PROGRAM MAIN
VAR CONSTANT
    cInitSource			: ST_MA_MultiArray_InitPars 
							:= ( eTypeCode := eMA_TypeCode_LREAL, nDims := 2, aDimSizes := [cChannels, cBufferLength]);
END_VAR

VAR
	(* Input *)	
	nInputSelection			: UDINT := 1;						// Switch between hardware and function generator	
	nSample					: UDINT;							// local variable
	// Hardware
	aEl3632Ch1 AT %I*		: ARRAY[1..cOversamples] OF INT;	// Input from hardware e.g. EL3632 ch1
	aEl3632Ch2 AT %I*		: ARRAY[1..cOversamples] OF INT;	// Input from hardware e.g. EL3632 ch2
	// Function generator
	fbFunctionGenerator1	: FB_FunctionGenerator;				// Signal Generator, ch1
	fSetFrequency1			: LREAL := 400;						// Hz
	fSetAmplitude1			: LREAL := 4;						// peak amplitude of sin signal [m/s^2]
	fbFunctionGenerator2	: FB_FunctionGenerator;				// Signal Generator, ch2
	fSetFrequency2			: LREAL := 35;						// Hz
	fSetAmplitude2			: LREAL := 4;						// peak amplitude of sin signal	[m/s^2]	
	fAmplitudeNoise         : LREAL;
	// additive noise for generated signals
	fbRand					: DRAND;                          	// random number generator
	fRandomNumber			: LREAL;							// value of noise
	fVar					: LREAL := 15;						// variance of added noise
		
	(* Input from aBuffer to fbSource *)
	aBuffer				: ARRAY[1..cChannels] OF ARRAY[1..cOversamples] OF LREAL;						
	fbSource			: FB_CMA_Source :=(	stInitPars := cInitSource, nOwnID := eID_Source, aDestIDs := [eID_IntegratedRMS]);
										
	(* From fbSink to aRMSResult *)	
	aRMSResult   		: ARRAY[1..cChannels] OF ARRAY[0..cOrderRMS] OF LREAL;	// Copy result
	fbIntRMS_Sink		: FB_CMA_Sink := (nOwnID := eID_IntegratedRMS_Sink);
	
	(* From fbMean_Sink to aRMSMean *)
	aRMSMean	    	: ARRAY[1..cChannels] OF ARRAY[0..cOrderRMS] OF LREAL;	// Copy result
	fbMean_Sink			: FB_CMA_Sink := (nOwnID := eID_EmpiricalMean_Sink);

	(* From fbStd_Sink to aRMSStd *)
	aRMSStd	    		: ARRAY[1..cChannels] OF ARRAY[0..cOrderRMS] OF LREAL;	// Copy result
	fbStd_Sink			: FB_CMA_Sink := (nOwnID := eID_EmpiricalStd_Sink);
	
	(* From fbClass_Sink to aClass *)	
	aClass				: ARRAY[1..cChannels] OF ARRAY[0..cOrderRMS] OF DINT;	// Copy result									
	fbClass_Sink		: FB_CMA_Sink := (nOwnID := eID_Classify_Sink);		
	
	(* Classify calculated RMS values *)
	nCountResults		: ULINT;
	bCalculate			: BOOL;
	bCalculateStat		: BOOL;
	bCalculateClass		: BOOL;
	ISOClassIs_Acc		: ARRAY[1..cChannels] OF E_IsoClass;
	ISOClassIs_Vel		: ARRAY[1..cChannels] OF E_IsoClass;
	ISOClassIs_Displ	: ARRAY[1..cChannels] OF E_IsoClass;
	
	(* little helper variables *)
	nChannel			: UDINT;
	Channel1			: ST_Channel;
	Channel2			: ST_Channel;
	
	(* output *)
	ISO_10816_Classification AT%Q* : E_IsoClass := E_IsoClass.N;

END_VAR

(* Generate input signals *)
MAIN.InputSignal();			

(* Call source to collect data *)
fbSource.Input2DStd(pDataIn 		:= ADR(aBuffer),
					nDataInSize 	:= SIZEOF(aBuffer), 
					eElementType	:= eMA_TypeCode_LREAL,
					nOptionPars		:= cCMA_Option_MarkInterruption ); 
IF fbSource.bError THEN
	fbErrHist.AddError(bErr:=TRUE, hrErrCode:=fbSource.hrErrorCode, sErrSource:='MAIN.fbSource.Input2DStd()'); // error monitoring
	// ToDo: if error
END_IF

(* Call Sinks to get results back to this task *)
MAIN.CallSinks();

(* Calculate results, i.e. determine classification *)
MAIN.CalculateResults();

ACTION CalculateResults:
// results of RMS calculation 
IF bCalculate THEN
	// channel 1
	Channel1.AccRMS   := aRMSResult[1][0];
	Channel1.VelRMS   := aRMSResult[1][1];
	Channel1.DispRMS  := aRMSResult[1][2];
	// channel 2
	Channel2.AccRMS   := aRMSResult[2][0];
	Channel2.VelRMS   := aRMSResult[2][1];
	Channel2.DispRMS  := aRMSResult[2][2];	
END_IF

// results of RMS statistics
IF bCalculateStat THEN
	// channel 1
	Channel1.AccMeanRMS				:= aRMSMean[1][0];
	Channel1.AccStdRMS				:= aRMSStd[1][0];
	Channel1.AccMeanPlusStdRms		:= Channel1.AccMeanRMS + Channel1.AccStdRMS;
	Channel1.AccMeanMinusStdRms		:= Channel1.AccMeanRMS - Channel1.AccStdRMS;
	Channel1.VelMeanRMS				:= aRMSMean[1][1];
	Channel1.VelStdRMS				:= aRMSStd[1][1];
	Channel1.VelMeanPlusStdRms		:= Channel1.VelMeanRMS + Channel1.VelStdRMS;
	Channel1.VelMeanMinusStdRms		:= Channel1.VelMeanRMS - Channel1.VelStdRMS;
	Channel1.DispMeanRMS			:= aRMSMean[1][2];
	Channel1.DispStdRMS				:= aRMSStd[1][2];
	Channel1.DispMeanPlusStdRms		:= Channel1.DispMeanRMS + Channel1.DispStdRMS;
	Channel1.DispMeanMinusStdRms	:= Channel1.DispMeanRMS - Channel1.DispStdRMS;
	
	// channel 2
	Channel2.AccMeanRMS				:= aRMSMean[2][0];
	Channel2.AccStdRMS				:= aRMSStd[2][0];
	Channel2.AccMeanPlusStdRms		:= Channel2.AccMeanRMS + Channel2.AccStdRMS;
	Channel2.AccMeanMinusStdRms		:= Channel2.AccMeanRMS - Channel2.AccStdRMS;
	Channel2.VelMeanRMS				:= aRMSMean[2][1];
	Channel2.VelStdRMS				:= aRMSStd[2][1];
	Channel2.VelMeanPlusStdRms		:= Channel2.VelMeanRMS + Channel2.VelStdRMS;
	Channel2.VelMeanMinusStdRms		:= Channel2.VelMeanRMS - Channel2.VelStdRMS;
	Channel2.DispMeanRMS			:= aRMSMean[2][2];
	Channel2.DispStdRMS				:= aRMSStd[2][2];
	Channel2.DispMeanPlusStdRms		:= Channel2.DispMeanRMS + Channel2.DispStdRMS;
	Channel2.DispMeanMinusStdRms	:= Channel2.DispMeanRMS - Channel2.DispStdRMS;
END_IF

// results of classification
IF bCalculateClass THEN
	nCountResults := nCountResults + 1;
	
	// do for each channel, shift classification results, i.e. convert range [-2..cMaxClasses-1] to [0..cMaxClasses+1]
	FOR nChannel := 1 TO cChannels DO
		ISOClassIs_Acc[nChannel]	:= DINT_TO_UDINT(aClass[nChannel][0] + 2);
		ISOClassIs_Vel[nChannel]	:= DINT_TO_UDINT(aClass[nChannel][1] + 2);
		ISOClassIs_Displ[nChannel]	:= DINT_TO_UDINT(aClass[nChannel][2] + 2);
	END_FOR
	
	// according to ISO 10816-3 select worst case 		
	ISO_10816_Classification := E_IsoClass.A;
	FOR  nChannel := 1 TO cChannels DO
		IF ISOClassIs_Acc[nChannel] > ISO_10816_Classification THEN
			ISO_10816_Classification := ISOClassIs_Acc[nChannel];
		END_IF
		IF ISOClassIs_Vel[nChannel] > ISO_10816_Classification THEN
			ISO_10816_Classification := ISOClassIs_Vel[nChannel];
		END_IF
		IF ISOClassIs_Displ[nChannel] > ISO_10816_Classification THEN
			ISO_10816_Classification := ISOClassIs_Displ[nChannel];
		END_IF
	END_FOR;

END_IF
END_ACTION

ACTION CallSinks:
(* Push results to sink *)
fbIntRMS_Sink.Output2DStd(	pDataOut 		:= ADR(aRMSResult), 
							nDataOutSize 	:= SIZEOF(aRMSResult), 
							eElementType 	:= eMA_TypeCode_LREAL, 
							nOptionPars		:= 0,
							bNewResult		=> bCalculate);
IF fbIntRMS_Sink.bError THEN
	fbErrHist.AddError(bErr:=TRUE, hrErrCode:=fbIntRMS_Sink.hrErrorCode, sErrSource:='MAIN.fbIntRMS_Sink.Output2DStd()'); // error monitoring
	// ToDo: if error
END_IF

(* Sink of mean of RMS *)
fbMean_Sink.Output2DStd(	pDataOut 		:= ADR(aRMSMean), 
							nDataOutSize 	:= SIZEOF(aRMSMean), 
							eElementType 	:= eMA_TypeCode_LREAL, 
							nOptionPars		:= 0,
							bNewResult		=> bCalculateStat);
IF fbMean_Sink.bError THEN
	fbErrHist.AddError(bErr:=TRUE, hrErrCode:=fbMean_Sink.hrErrorCode, sErrSource:='MAIN.fbMean_Sink.Output2DStd()'); // error monitoring
	// ToDo: if error
END_IF

(* Sink of standard deviation of RMS *)
fbStd_Sink.Output2DStd(	pDataOut 		:= ADR(aRMSStd), 
						nDataOutSize 	:= SIZEOF(aRMSStd), 
						eElementType 	:= eMA_TypeCode_LREAL, 
						nOptionPars		:= 0,
						bNewResult		=> bCalculateStat);
IF fbStd_Sink.bError THEN
	fbErrHist.AddError(bErr:=TRUE, hrErrCode:=fbStd_Sink.hrErrorCode, sErrSource:='MAIN.fbStd_Sink.Output2DStd()'); // error monitoring
	// ToDo: if error
END_IF

(* Sink classification *)
fbClass_Sink.Output2DStd(	pDataOut 		:= ADR(aClass), 
							nDataOutSize 	:= SIZEOF(aClass), 
							eElementType 	:= eMA_TypeCode_INT32, 
							nOptionPars		:= 0,
							bNewResult		=> bCalculateClass);
IF fbClass_Sink.bError THEN
	fbErrHist.AddError(bErr:=TRUE, hrErrCode:=fbClass_Sink.hrErrorCode, sErrSource:='MAIN.fbClass_Sink.Output2DStd()'); // error monitoring
	// ToDo: if error
END_IF
END_ACTION

ACTION InputSignal:
// choose between real input and function generator with added noise
CASE nInputSelection OF
	0:  (* input from EL3632 *)
		FOR nSample := 1 TO cOversamples DO
			aBuffer[1][nSample] := cScale*INT_TO_LREAL(aEl3632Ch1[nSample]); // convert from Volts to acceleration in m/s^2
			aBuffer[2][nSample] := cScale*INT_TO_LREAL(aEl3632Ch2[nSample]);
		END_FOR 
	1:  (* signal generator *)		
		fbFunctionGenerator1(	fFrequency 	:= fSetFrequency1,
								fAmplitude 	:= fSetAmplitude1,
								eFunction 	:= E_FunctionType.Sine,
								aSignal		:= aBuffer[1]);	
		fbFunctionGenerator2(	fFrequency 	:= fSetFrequency2,
								fAmplitude 	:= fSetAmplitude2,
								eFunction 	:= E_FunctionType.Sine,
								aSignal		:= aBuffer[2]);	
		// Input signal with disturbance
		FOR nSample := 1 TO cOversamples DO	
			// Random number generator	
			fbRand(Seed := 	1000, Num => fRandomNumber);			
			aBuffer[1][nSample] := aBuffer[1][nSample] + fVar*fRandomNumber;
			fbRand(Seed := 	1000, Num => fRandomNumber);			
			aBuffer[2][nSample] := aBuffer[2][nSample] + 1.5*fVar*fRandomNumber;	// more noise on channel 2
		END_FOR									
END_CASE
END_ACTION

END_PROGRAM
